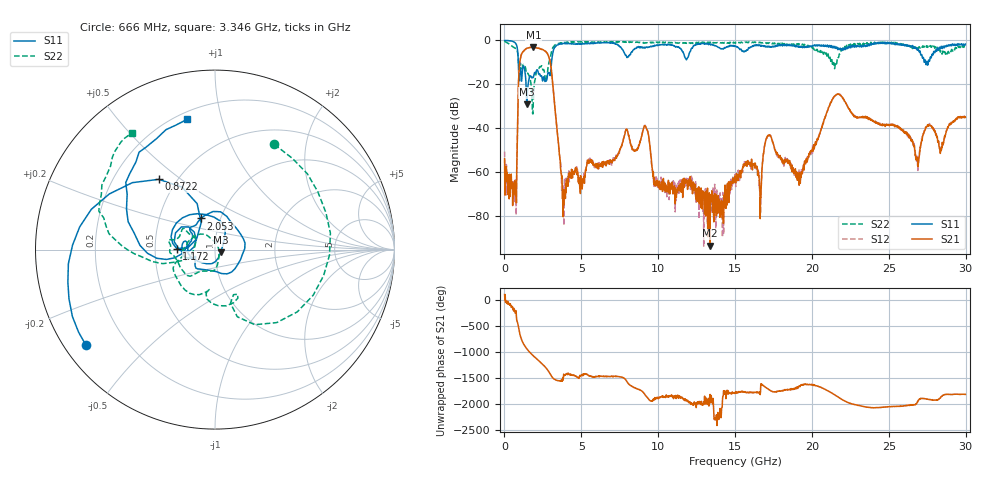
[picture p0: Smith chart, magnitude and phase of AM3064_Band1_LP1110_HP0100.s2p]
# Hz S DB R 50.0
!freq dBS11 angS11 dBS21 angS21 dBS12 angS12 dBS22 angS22
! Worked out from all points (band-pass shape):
!   1600 points, 10 MHz to 29.98 GHz, reference 50 ohm
!   highest |S21| = -3.14 dB at 1.884 GHz (marker M1); lowest = -93.7 dB at 13.37 GHz (marker M2)
!   |S21| within 3 dB of the highest: 1.118 GHz to 2.798 GHz (1.68 GHz wide, 85.8 % of centre)
!   lowest |S11| = -29.1 dB at 1.453 GHz (marker M3), VSWR 1.07, Z = 53.2 - j1.64 ohm
!   |S11| at or under -10 dB: 902.3 MHz to 3.061 GHz (2.159 GHz wide, 109 % of centre); 27.39235 GHz to 27.45934 GHz (66.99 MHz wide, 0.244 % of centre); 27.48974 GHz to 27.56345 GHz (73.72 MHz wide, 0.268 % of centre)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
!   |S22| runs from -33.6 to -0.4 dB; largest |S21 - S12| = 0.011
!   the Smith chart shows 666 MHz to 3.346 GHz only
!   S11 on the Smith chart (normalised r, x): 666 MHz: 0.06, -0.33; 872.2 MHz: 0.40, +0.42; 1.172 GHz: 0.65, +0.01; 2.053 GHz: 0.81, +0.29; 3.346 GHz: 0.24, +0.78
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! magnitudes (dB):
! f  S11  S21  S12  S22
! 10 MHz  0.0  -54.0  -50.7  -0.4
! 666 MHz  -1.0  -64.0  -64.3  -3.4
! 872.2 MHz  -6.0  -31.0  -30.9  -6.5
! 1.172 GHz  -13.4  -5.5  -5.4  -12.1
! 1.453 GHz  -29.1  -3.6  -3.6  -15.2
! 1.884 GHz  -16.7  -3.1  -3.2  -26.1
! 2.053 GHz  -14.4  -3.4  -3.3  -15.0
! 2.897 GHz  -14.7  -7.7  -7.7  -10.0
! 3.346 GHz  -2.6  -35.4  -35.4  -2.0
! 3.852 GHz  -1.4  -75.2  -75.9  -1.1
! 5.015 GHz  -1.6  -67.5  -64.8  -0.6
! 9.157 GHz  -3.5  -39.1  -38.7  -1.1
! 10 GHz  -2.2  -66.6  -65.3  -0.9
! 13.37 GHz  -1.7  -93.7  -85.7  -0.9
! 15 GHz  -2.8  -63.1  -61.1  -1.3
! 16.62 GHz  -2.0  -67.9  -67.9  -0.8
! 17.18 GHz  -2.8  -43.5  -43.0  -1.4
! 19.99 GHz  -2.8  -50.5  -50.2  -3.1
! 21.64 GHz  -3.4  -24.5  -24.7  -8.6
! 25 GHz  -1.0  -38.7  -38.7  -1.1
! 26.85 GHz  -4.5  -54.1  -54.3  -2.8
! 29.98 GHz  -1.7  -35.0  -35.1  -2.8
